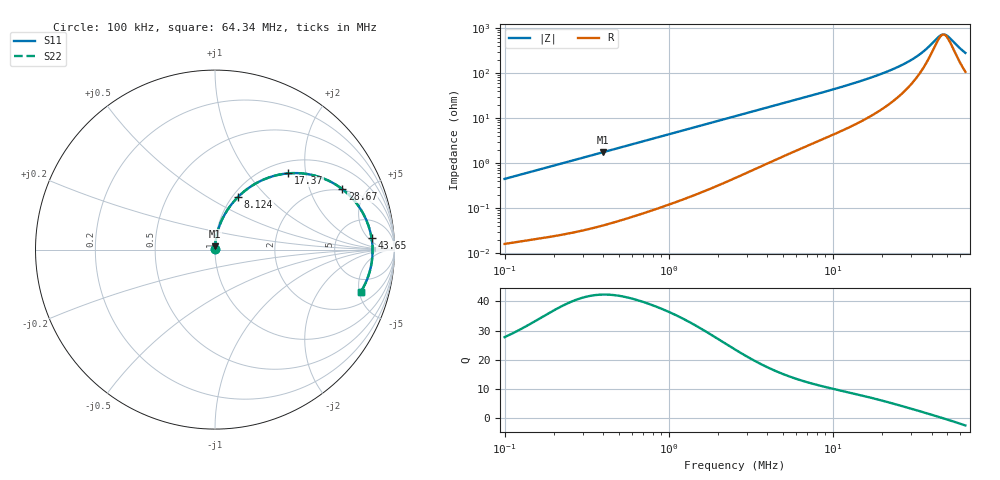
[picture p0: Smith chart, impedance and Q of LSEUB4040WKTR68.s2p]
! LSEUB4040WKTR68  S-PARAMETER MODEL  ( Standard Model )
! Model Generated by TAIYO YUDEN Corporation (http://www.ty-top.com)
! Version 1.0
! TAIYO YUDEN Control No. 20230502
! Copyright(c) 2023 TAIYO YUDEN CO.,LTD. All Rights Reserved.
! Product Description (link to TY-COMPAS)
! https://ds.yuden.co.jp/TYCOMPAS/or/detail?pn=LSEUB4040WKTR68M&u=M
! Products Name : Inductors
! Characteristics :
!  Inductance : 0.68 [uH] , SRF(min) : - [Hz] , DC Resistance(max) : 0.009 [Ohm]
!  Rated Current : Saturation  11000 [mA] , Temp Rise  8400 [mA] (40 [degC])
!  Case Size : 4.0 x 4.0 / 0.157 x 0.157 [mm/inch] , Thickness : 2.0 / 0.079 [mm/inch]
!  (Conditions: Temperature = 25 [degC] , DC Bias Current = 0 [A])
! External Node Assignments :
!  1  o---GGG---o  2
! GND o---------o GND
! Frequency Range : 0.1MHz  -  64.339822MHz  [ 402 STEP ]
# MHz S RI R 50
! Freq[MHz].  S11 Real  S11 Imag  S21 Real  S21 Imag  S12 Real  S12 Imag  S22 Real  S22 Imag
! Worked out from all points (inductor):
!   401 points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, 100 kHz to 64.34 MHz, reference 50 ohm
!   read as one part in series: L = 707 nH near 103.3 kHz
!   highest Q = 42.3 at 395.2 kHz (marker M1), where L = 699 nH
!   self-resonance near 47.27 MHz
!   S11 on the Smith chart (normalised r, x): 100 kHz: 1.00, +0.01; 8.124 MHz: 1.06, +0.69; 17.37 MHz: 1.23, +1.60; 28.67 MHz: 1.94, +3.40; 43.65 MHz: 12, +6; 64.34 MHz: 3.14, -5.19
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0.1  0.000181 0.00446  0.9998 -0.00446  0.9998 -0.00446  0.000181 0.00446
0.295407  0.000485 0.013  0.9995 -0.013  0.9995 -0.013  0.000485 0.013
0.395186  0.00071 0.0173  0.9993 -0.0173  0.9993 -0.0173  0.00071 0.0173
0.872651  0.00244 0.0379  0.9976 -0.0379  0.9976 -0.0379  0.00244 0.0379
2.53653  0.0163 0.1071  0.9837 -0.1071  0.9837 -0.1071  0.0163 0.1071
4.688625  0.0499 0.1882  0.9501 -0.1882  0.9501 -0.1882  0.0499 0.1882
7.493079  0.1122 0.2763  0.8878 -0.2763  0.8878 -0.2763  0.1122 0.2763
8.123932  0.1284 0.2933  0.8716 -0.2933  0.8716 -0.2933  0.1284 0.2933
11.97499  0.2387 0.3749  0.7613 -0.3749  0.7613 -0.3749  0.2387 0.3749
17.36851  0.4086 0.4248  0.5914 -0.4248  0.5914 -0.4248  0.4086 0.4248
22.13506  0.5515 0.4133  0.4485 -0.4133  0.4485 -0.4133  0.5515 0.4133
25.19128  0.6319 0.3843  0.3681 -0.3843  0.3681 -0.3843  0.6319 0.3843
28.66948  0.7095 0.3368  0.2905 -0.3368  0.2905 -0.3368  0.7095 0.3368
32.10467  0.7706 0.2795  0.2294 -0.2795  0.2294 -0.2795  0.7706 0.2795
35.37492  0.8146 0.2197  0.1854 -0.2197  0.1854 -0.2197  0.8146 0.2197
38.35319  0.8436 0.1633  0.1564 -0.1633  0.1564 -0.1633  0.8436 0.1633
43.64867  0.8723 0.0642  0.1277 -0.0642  0.1277 -0.0642  0.8723 0.0642
46.5646  0.8776 0.0122  0.1224 -0.0122  0.1224 -0.0122  0.8776 0.0122
48.87868  0.8775 -0.0271  0.1225 0.0271  0.1225 0.0271  0.8775 -0.0271
51.30776  0.8738 -0.0662  0.1262 0.0662  0.1262 0.0662  0.8738 -0.0662
60.31079  0.8366 -0.1906  0.1634 0.1906  0.1634 0.1906  0.8366 -0.1906
64.33982  0.8121 -0.2357  0.1879 0.2357  0.1879 0.2357  0.8121 -0.2357
